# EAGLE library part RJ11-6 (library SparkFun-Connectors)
RJ11 Jack - 6 pin Commonly found on CAT3 devices and some Microchip programmers. Here is the connector we sell at SparkFun: RJ11 6-Pin Connector (PRT-00132) Datasheet It is used on this SparkFun product: SparkFun Weather Shield (DEV-12081) Weather Meters (SEN-08942)
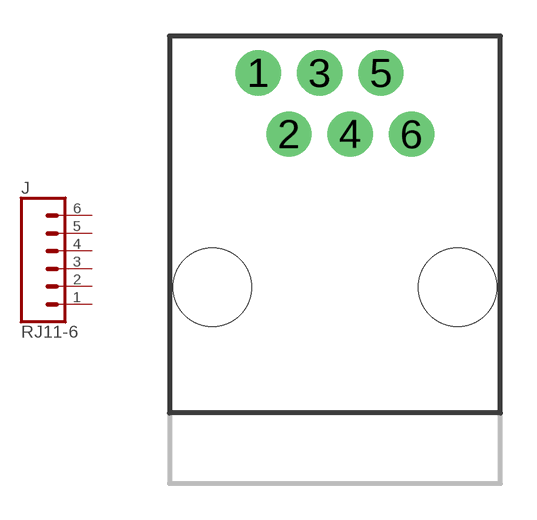
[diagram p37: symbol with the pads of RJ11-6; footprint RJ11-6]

Designator prefix J

## RJ11-6 (PROD_ID: CONN-08590; SF_ID: PRT-00132; VALUE: RJ11)  [RJ11-6]
1  1  pas
2  2  pas
3  3  pas
4  4  pas
5  5  pas
6  6  pas

## Footprint RJ11-6 (pad centres in mm)
RJ11 6-Pin Socket with PCB Mounting Post Specifications: Pin count: 6 Datasheet referenced for footprint Example device(s): RJ11-6
drill 1.016 pad 1.88: 1 -3.175,8.89; 2 -1.905,6.35; 3 -0.635,8.89; 4 0.635,6.35; 5 1.905,8.89; 6 3.175,6.35
hole 3.251 at -5.08,0
hole 3.251 at 5.08,0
